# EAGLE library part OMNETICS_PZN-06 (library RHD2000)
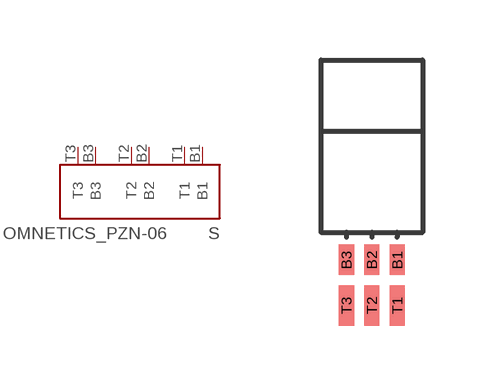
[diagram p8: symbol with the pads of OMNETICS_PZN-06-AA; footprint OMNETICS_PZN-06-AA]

Designator prefix S

## OMNETICS_PZN-06_SMD  [OMNETICS_PZN-06-AA]
B1  B1
B2  B2
B3  B3
T1  T1
T2  T2
T3  T3

## Footprint OMNETICS_PZN-06-AA (pad centres in mm)
smd 0.381 x 0.762: B1 0.635,-1.016; B2 0,-1.016; B3 -0.635,-1.016
smd 0.381 x 1.016: T1 0.635,-2.159; T2 0,-2.159; T3 -0.635,-2.159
